| TEXAS INSTRUMENTS INCORPORATED
| Standard Linear and Logic Group
| IBIS Model of SN74AHC16240
| 16-BIT BUFFERS/DRIVERS WITH 3-STATE OUTPUTS
| This file contains package information for the following:
|  TSSOP 48-pin (DGG) package as [Component] AHC16240_DGG
|  TVSOP 48-pin (DGV) package as [Component] AHC16240_DGV
|  SSOP 48-pin (DL) package as [Component] AHC16240_DL
| This device can be powered at the following Vccs:
|  5 volt Vcc
|  3.3 volt Vcc
|  2.2 volt Vcc
| This file provides unique models under the [Model Selector] for each Vcc.
| For operation at a specific Vcc, select the appropriate model after each
| [Model Selector] keyword.
[IBIS Ver]   3.2
[Comment char]  |_char
[File Name]   sn74ahc16240.ibs
[File Rev]   1.1 | x_die
[Date]   May 27, 2002
[Source]   Data created from TI-SPICE simulations at TI-SLL.
[Notes]   The following is an IBIS list for the SN74AHC16240.
   Please contact sllibis@ti.com with questions and
   comments concerning SLL IBIS models.
[Disclaimer] Property of Texas Instruments Incorporated.  Unauthorized
   reproduction and/or distribution is strictly prohibited.
   This product is protected under copyright law.
   Created  2002, (C) Copyright  2002, Texas Instruments
   Incorporated, All Rights Reserved
   UNLESS THERE IS A SIGNED, WRITTEN AGREEMENT TO THE
   CONTRARY, TEXAS INSTRUMENTS (TI) IS PROVIDING THE IBIS
   MODELS  AND WITHOUT ANY WARRANTY, EXPRESSED OR
   IMPLIED.  TI assumes no liability for:
   1) the accuracy of the IBIS models provided to your
   company;
   2) the proper functioning of these IBIS Models in your
   design or for any resulting applications; or
   3) infringement of patents, copyrights or intellectual
   property rights resulting from your use of these IBIS
   models.
   TI provides IBIS Models as a service to our customers.
   You and your company shall not distribute, sell or give
   these models to anyone else without prior written
   permission from TI.
   TI reserves the right to make changes to our products or
   to discontinue any semiconductor product or service
   without notice, and advises our customers to obtain the
   latest version of relevant information to verify, before
   placing orders, that the information being relied on is
   current.
   Please be aware that your receipt and use of the IBIS
   information provided shall serve as acceptance of these
   terms and conditions.  If you do not accept these terms,
   you should return or destroy the IBIS models and any
   other accompanying information immediately.
| Component AHC16240_DGG 48-pin TSSOP
[Component]   AHC16240_DGG
[Manufacturer]   Texas Instruments, Inc.
[Package]
|   typ   min   max
R_pkg   4.400e-02   3.800e-02   5.100e-02
L_pkg   3.019e-09   2.486e-09   4.099e-09
C_pkg   5.070e-13   3.340e-13   8.090e-13
[Pin]   signal_name   model_name   R_pin   L_pin   C_pin
1   1NOE   AHC16240_OE   4.100e-02   4.017e-09   7.590e-13
2   1Y1   AHC16240_OUT   4.200e-02   3.737e-09   7.920e-13
3   1Y2   AHC16240_OUT   4.200e-02   3.480e-09   6.610e-13
4   GND   GND   3.800e-02   3.131e-09   5.750e-13
5   1Y3   AHC16240_OUT   4.700e-02   3.122e-09   5.660e-13
6   1Y4   AHC16240_OUT   4.300e-02   2.948e-09   5.040e-13
7   VCC   POWER   4.500e-02   2.845e-09   3.970e-13
8   2Y1   AHC16240_OUT   4.900e-02   2.835e-09   3.940e-13
9   2Y2   AHC16240_OUT   4.800e-02   2.715e-09   3.780e-13
10   GND   GND   5.000e-02   2.664e-09   3.630e-13
11   2Y3   AHC16240_OUT   5.000e-02   2.585e-09   3.480e-13
12   2Y4   AHC16240_OUT   4.900e-02   2.550e-09   3.370e-13
13   3Y1   AHC16240_OUT   4.900e-02   2.541e-09   3.360e-13
14   3Y2   AHC16240_OUT   5.000e-02   2.574e-09   3.480e-13
15   GND   GND   4.900e-02   2.618e-09   3.590e-13
16   3Y3   AHC16240_OUT   4.600e-02   2.671e-09   3.750e-13
17   3Y4   AHC16240_OUT   4.500e-02   2.754e-09   3.890e-13
18   VCC   POWER   4.400e-02   2.823e-09   4.500e-13
19   4Y1   AHC16240_OUT   4.200e-02   2.968e-09   5.030e-13
20   4Y2   AHC16240_OUT   5.100e-02   3.108e-09   5.350e-13
21   GND   GND   4.200e-02   3.175e-09   5.870e-13
22   4Y3   AHC16240_OUT   4.100e-02   3.449e-09   6.780e-13
23   4Y4   AHC16240_OUT   4.400e-02   3.766e-09   8.040e-13
24   4NOE   AHC16240_OE   4.300e-02   4.065e-09   7.610e-13
25   3NOE   AHC16240_OE   4.100e-02   3.994e-09   7.570e-13
26   4A4   AHC16240_IN   3.900e-02   3.649e-09   7.890e-13
27   4A3   AHC16240_IN   3.800e-02   3.362e-09   6.600e-13
28   GND   GND   3.800e-02   3.082e-09   5.740e-13
29   4A2   AHC16240_IN   4.400e-02   2.990e-09   5.220e-13
30   4A1   AHC16240_IN   4.100e-02   2.917e-09   4.950e-13
31   VCC   POWER   4.300e-02   2.820e-09   4.480e-13
32   3A4   AHC16240_IN   4.300e-02   2.699e-09   3.850e-13
33   3A3   AHC16240_IN   4.500e-02   2.628e-09   3.720e-13
34   GND   GND   4.600e-02   2.556e-09   3.560e-13
35   3A2   AHC16240_IN   4.600e-02   2.495e-09   3.440e-13
36   3A1   AHC16240_IN   4.700e-02   2.487e-09   3.340e-13
37   2A4   AHC16240_IN   4.700e-02   2.490e-09   3.350e-13
38   2A3   AHC16240_IN   4.600e-02   2.486e-09   3.430e-13
39   GND   GND   4.500e-02   2.566e-09   3.560e-13
40   2A2   AHC16240_IN   4.400e-02   2.639e-09   3.740e-13
41   2A1   AHC16240_IN   4.300e-02   2.701e-09   3.860e-13
42   VCC   POWER   4.300e-02   2.817e-09   4.500e-13
43   1A4   AHC16240_IN   4.100e-02   2.935e-09   5.010e-13
44   1A3   AHC16240_IN   4.700e-02   3.035e-09   5.290e-13
45   GND   GND   4.300e-02   3.171e-09   5.890e-13
46   1A2   AHC16240_IN   4.000e-02   3.415e-09   6.820e-13
47   1A1   AHC16240_IN   4.300e-02   3.741e-09   8.090e-13
48   2NOE   AHC16240_OE   4.400e-02   4.099e-09   7.640e-13
| Component AHC16240_DGV 48-pin TVSOP
[Component]   AHC16240_DGV
[Manufacturer]   Texas Instruments, Inc.
[Package]
|   typ   min   max
R_pkg   7.000e-02   4.900e-02   8.500e-02
L_pkg   3.013e-09   2.743e-09   3.408e-09
C_pkg   3.710e-13   2.940e-13   5.110e-13
[Pin]   signal_name   model_name   R_pin   L_pin   C_pin
1   1NOE   AHC16240_OE   4.900e-02   3.393e-09   4.970e-13
2   1Y1   AHC16240_OUT   6.000e-02   3.250e-09   5.020e-13
3   1Y2   AHC16240_OUT   7.700e-02   3.310e-09   4.510e-13
4   GND   GND   8.500e-02   3.299e-09   4.040e-13
5   1Y3   AHC16240_OUT   8.300e-02   3.136e-09   3.600e-13
6   1Y4   AHC16240_OUT   7.700e-02   3.019e-09   3.630e-13
7   VCC   POWER   6.500e-02   2.882e-09   3.490e-13
8   2Y1   AHC16240_OUT   6.600e-02   2.829e-09   3.140e-13
9   2Y2   AHC16240_OUT   6.700e-02   2.796e-09   3.140e-13
10   GND   GND   6.900e-02   2.754e-09   3.080e-13
11   2Y3   AHC16240_OUT   7.000e-02   2.753e-09   3.010e-13
12   2Y4   AHC16240_OUT   7.100e-02   2.745e-09   2.940e-13
13   3Y1   AHC16240_OUT   7.000e-02   2.744e-09   2.940e-13
14   3Y2   AHC16240_OUT   7.000e-02   2.754e-09   3.010e-13
15   GND   GND   6.900e-02   2.754e-09   3.080e-13
16   3Y3   AHC16240_OUT   6.700e-02   2.796e-09   3.140e-13
17   3Y4   AHC16240_OUT   6.600e-02   2.829e-09   3.140e-13
18   VCC   POWER   6.500e-02   2.883e-09   3.500e-13
19   4Y1   AHC16240_OUT   7.500e-02   3.014e-09   3.630e-13
20   4Y2   AHC16240_OUT   8.000e-02   3.128e-09   3.580e-13
21   GND   GND   8.400e-02   3.295e-09   4.030e-13
22   4Y3   AHC16240_OUT   7.800e-02   3.311e-09   4.520e-13
23   4Y4   AHC16240_OUT   6.200e-02   3.259e-09   5.010e-13
24   4NOE   AHC16240_OE   5.200e-02   3.404e-09   4.960e-13
25   3NOE   AHC16240_OE   5.300e-02   3.397e-09   5.050e-13
26   4A4   AHC16240_IN   6.200e-02   3.249e-09   5.110e-13
27   4A3   AHC16240_IN   7.700e-02   3.308e-09   4.530e-13
28   GND   GND   8.200e-02   3.289e-09   4.030e-13
29   4A2   AHC16240_IN   7.800e-02   3.121e-09   3.590e-13
30   4A1   AHC16240_IN   7.400e-02   3.010e-09   3.630e-13
31   VCC   POWER   6.500e-02   2.883e-09   3.490e-13
32   3A4   AHC16240_IN   6.700e-02   2.829e-09   3.140e-13
33   3A3   AHC16240_IN   6.700e-02   2.795e-09   3.140e-13
34   GND   GND   6.900e-02   2.753e-09   3.070e-13
35   3A2   AHC16240_IN   7.000e-02   2.753e-09   3.010e-13
36   3A1   AHC16240_IN   7.000e-02   2.743e-09   2.940e-13
37   2A4   AHC16240_IN   7.000e-02   2.743e-09   2.940e-13
38   2A3   AHC16240_IN   7.000e-02   2.753e-09   3.010e-13
39   GND   GND   6.900e-02   2.754e-09   3.070e-13
40   2A2   AHC16240_IN   6.800e-02   2.797e-09   3.140e-13
41   2A1   AHC16240_IN   6.700e-02   2.830e-09   3.140e-13
42   VCC   POWER   6.400e-02   2.880e-09   3.490e-13
43   1A4   AHC16240_IN   7.200e-02   3.004e-09   3.620e-13
44   1A3   AHC16240_IN   7.800e-02   3.121e-09   3.590e-13
45   GND   GND   8.400e-02   3.296e-09   4.030e-13
46   1A2   AHC16240_IN   7.700e-02   3.308e-09   4.510e-13
47   1A1   AHC16240_IN   6.200e-02   3.258e-09   4.990e-13
48   2NOE   AHC16240_OE   5.300e-02   3.408e-09   4.940e-13
| Component AHC16240_DL 48-pin SSOP
[Component]   AHC16240_DL
[Manufacturer]   Texas Instruments, Inc.
[Package]
|   typ   min   max
R_pkg   4.800e-02   3.800e-02   5.300e-02
L_pkg   6.046e-09   5.084e-09   7.968e-09
C_pkg   8.130e-13   5.690e-13   1.157e-12
[Pin]   signal_name   model_name   R_pin   L_pin   C_pin
1   1NOE   AHC16240_OE   4.600e-02   7.968e-09   1.017e-12
2   1Y1   AHC16240_OUT   4.400e-02   7.299e-09   1.157e-12
3   1Y2   AHC16240_OUT   4.300e-02   6.765e-09   1.058e-12
4   GND   GND   4.100e-02   6.269e-09   9.330e-13
5   1Y3   AHC16240_OUT   3.800e-02   5.856e-09   8.290e-13
6   1Y4   AHC16240_OUT   4.600e-02   5.802e-09   7.900e-13
7   VCC   POWER   5.000e-02   5.656e-09   7.380e-13
8   2Y1   AHC16240_OUT   5.300e-02   5.500e-09   6.430e-13
9   2Y2   AHC16240_OUT   5.200e-02   5.304e-09   6.060e-13
10   GND   GND   5.300e-02   5.189e-09   5.830e-13
11   2Y3   AHC16240_OUT   5.100e-02   5.084e-09   5.690e-13
12   2Y4   AHC16240_OUT   5.300e-02   5.862e-09   8.330e-13
13   3Y1   AHC16240_OUT   5.300e-02   5.862e-09   8.330e-13
14   3Y2   AHC16240_OUT   5.100e-02   5.084e-09   5.690e-13
15   GND   GND   5.300e-02   5.189e-09   5.830e-13
16   3Y3   AHC16240_OUT   5.200e-02   5.304e-09   6.060e-13
17   3Y4   AHC16240_OUT   5.300e-02   5.500e-09   6.430e-13
18   VCC   POWER   5.000e-02   5.656e-09   7.380e-13
19   4Y1   AHC16240_OUT   4.600e-02   5.802e-09   7.900e-13
20   4Y2   AHC16240_OUT   3.800e-02   5.856e-09   8.290e-13
21   GND   GND   4.100e-02   6.269e-09   9.330e-13
22   4Y3   AHC16240_OUT   4.300e-02   6.765e-09   1.058e-12
23   4Y4   AHC16240_OUT   4.400e-02   7.299e-09   1.157e-12
24   4NOE   AHC16240_OE   4.600e-02   7.968e-09   1.017e-12
25   3NOE   AHC16240_OE   4.600e-02   7.968e-09   1.017e-12
26   4A4   AHC16240_IN   4.400e-02   7.299e-09   1.157e-12
27   4A3   AHC16240_IN   4.300e-02   6.765e-09   1.058e-12
28   GND   GND   4.100e-02   6.269e-09   9.330e-13
29   4A2   AHC16240_IN   3.800e-02   5.856e-09   8.290e-13
30   4A1   AHC16240_IN   4.600e-02   5.802e-09   7.900e-13
31   VCC   POWER   5.000e-02   5.656e-09   7.380e-13
32   3A4   AHC16240_IN   5.300e-02   5.500e-09   6.430e-13
33   3A3   AHC16240_IN   5.200e-02   5.304e-09   6.060e-13
34   GND   GND   5.300e-02   5.189e-09   5.830e-13
35   3A2   AHC16240_IN   5.100e-02   5.084e-09   5.690e-13
36   3A1   AHC16240_IN   5.300e-02   5.862e-09   8.330e-13
37   2A4   AHC16240_IN   5.300e-02   5.862e-09   8.330e-13
38   2A3   AHC16240_IN   5.100e-02   5.084e-09   5.690e-13
39   GND   GND   5.300e-02   5.189e-09   5.830e-13
40   2A2   AHC16240_IN   5.200e-02   5.304e-09   6.060e-13
41   2A1   AHC16240_IN   5.300e-02   5.500e-09   6.430e-13
42   VCC   POWER   5.000e-02   5.656e-09   7.380e-13
43   1A4   AHC16240_IN   4.600e-02   5.802e-09   7.900e-13
44   1A3   AHC16240_IN   3.800e-02   5.856e-09   8.290e-13
45   GND   GND   4.100e-02   6.269e-09   9.330e-13
46   1A2   AHC16240_IN   4.300e-02   6.765e-09   1.058e-12
47   1A1   AHC16240_IN   4.400e-02   7.299e-09   1.157e-12
48   2NOE   AHC16240_OE   4.600e-02   7.967e-09   1.017e-12
| Model AHC16240_IN
[Model Selector]   AHC16240_IN
AHC16240_IN_50   5 volt Vcc
AHC16240_IN_33   3.3 volt Vcc
AHC16240_IN_22   2.2 volt Vcc
| Model AHC16240_OE
[Model Selector]   AHC16240_OE
AHC16240_OE_50   5 volt Vcc
AHC16240_OE_33   3.3 volt Vcc
AHC16240_OE_22   2.2 volt Vcc
| Model AHC16240_OUT
[Model Selector]   AHC16240_OUT
AHC16240_OUT_50   5 volt Vcc
AHC16240_OUT_33   3.3 volt Vcc
AHC16240_OUT_22   2.2 volt Vcc
| Models and submodels in the file (9): AHC16240_IN_50 (Input), AHC16240_IN_33 (Input), AHC16240_IN_22 (Input), AHC16240_OE_50 (Input), AHC16240_OE_33 (Input), AHC16240_OE_22 (Input), AHC16240_OUT_50 (3-state), AHC16240_OUT_33 (3-state), AHC16240_OUT_22 (3-state)
